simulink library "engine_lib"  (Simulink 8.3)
settings: Solver=ode45  StartTime=0.0  StopTime=10.0  RelTol=1e-3
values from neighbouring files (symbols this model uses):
  engine = class_REVS_engine    [engine_2010_NA.m]    (also in engine_EGRB24_TDS.m)
libraries: general_lib x43, simulink x11, audit_lib x2

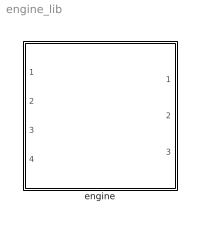
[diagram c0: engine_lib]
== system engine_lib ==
  engine : Subsystem

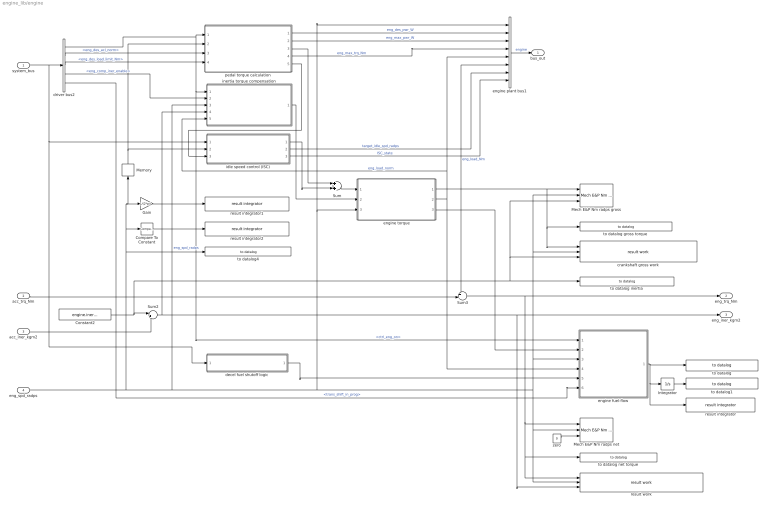
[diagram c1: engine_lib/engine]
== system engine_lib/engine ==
  system_bus : Inport
  acc_trq_Nm : Inport  Port=2
  acc_iner_kgm2 : Inport  Port=3
  eng_spd_radps : Inport  Port=4
  Compare To Constant : simulink/Logic and Bit Operations/Compare To Constant  relop=>  const=0  OutDataTypeStr=boolean  ZeroCross=off
  Constant2 : Constant  Value=engine.inertia_kgm2
  Gain : Gain  Gain=1/(2*pi)
  Integrator : Integrator
  Mech E&P Nm radps gross : audit_lib/Mech E&P Nm radps  base_name=engine.crankshaft_gross  VerboseSignal=REVS.verbose
  Mech E&P Nm radps net : audit_lib/Mech E&P Nm radps  base_name=engine.crankshaft  VerboseSignal=REVS.verbose
  Memory : Memory
  Sum : Sum
  Sum2 : Sum  Inputs=|++
  Sum3 : Sum  Inputs=++|
  crankshaft gross work : general_lib/result work  ResultSignalName=crankshaft_gross_pos_work_kJ
  decel fuel shutoff logic : Subsystem
  driver bus2 : BusSelector  OutputSignals=powertrain.control.ctrl_eng_on,powertrain.trans.ctrl.eng_des_acl_norm,powertrain.trans.ctrl.eng_des_load_limit_Nm,powertrain.trans.ctrl.eng_comp_iner_enable,powertrain.trans.ctrl.core_ctl.trans_shift_in_prog
  engine fuel-flow : Subsystem
  engine plant bus1 : BusCreator  Inputs=8
  engine torque : Subsystem
  idle speed control (ISC) : Subsystem
  inertia torque compensation : Subsystem
  pedal torque calculation : Subsystem
  result integrator : general_lib/result integrator  ResultSignalName=fuel_consumed_g  ResultBaseName=''
  result integrator1 : general_lib/result integrator  ResultSignalName=engine_revolutions  ResultBaseName=''
  result integrator2 : general_lib/result integrator  ResultSignalName=engine_running_time_secs  ResultBaseName=''
  result work : general_lib/result work  ResultSignalName=crankshaft_output_pos_work_kJ
  to datalog : general_lib/to datalog  VarName=engine__fuel_rate_gps  WorkspaceName=datalog__engine__fuel_rate_gps  VerboseLevel=0  VerboseSignal=REVS.verbose
  to datalog gross torque : general_lib/to datalog  VarName=engine__crankshaft_gross_torque_Nm  WorkspaceName=datalog__engine__crankshaft_gross_torque_Nm  VerboseLevel=0  VerboseSignal=REVS.verbose
  to datalog inertia : general_lib/to datalog  VarName=engine__crankshaft_gross_inertia_kgm2  WorkspaceName=datalog__engine__crankshaft_gross_inertia_kgm2  VerboseLevel=0  VerboseSignal=REVS.verbose
  to datalog net torque : general_lib/to datalog  VarName=engine__crankshaft_torque_Nm  WorkspaceName=datalog__engine__crankshaft_torque_Nm  VerboseLevel=0  VerboseSignal=REVS.verbose
  to datalog1 : general_lib/to datalog  VarName=engine__fuel_consumed_g  WorkspaceName=datalog__engine__fuel_consumed_g  VerboseLevel=0  VerboseSignal=REVS.verbose
  to datalog4 : general_lib/to datalog  VarName=engine__crankshaft_speed_radps  WorkspaceName=datalog__engine__crankshaft_speed_radps  VerboseLevel=0  VerboseSignal=REVS.verbose
  zero : Constant  Value=0
  bus_out : Outport
  eng_trq_Nm : Outport  Port=2
  eng_iner_kgm2 : Outport  Port=3
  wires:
  idle speed control (ISC)/2(target_idle_spd_radps) -> engine plant bus1/7  "target_idle_spd_radps"
  decel fuel shutoff logic/1(eng_decel_fuel_cut_disable) -> engine fuel-flow/5(eng_decel_fuel_cut_disable)
  engine torque/3(eng_fuel_trq_Nm) -> engine fuel-flow/2(eng_trq_Nm)
  acc_trq_Nm/1 -> Sum3/2
  pedal torque calculation/2(current_max_pwr_W) -> engine plant bus1/3  "eng_max_pwr_W"
  pedal torque calculation/1(des_pwr_W) -> engine plant bus1/2  "eng_des_pwr_W"
  acc_iner_kgm2/1 -> Sum2/2
  driver bus2/2 -> pedal torque calculation/3(eng_des_acl_norm)  "<eng_des_acl_norm>"
  engine plant bus1/1 -> bus_out/1  "engine"
  pedal torque calculation/3(des_trq_Nm) -> Sum/1
  idle speed control (ISC)/1(trq_out_Nm) -> Sum/2
  Sum/1 -> engine torque/1(eng_slow_trq_Nm)
  system_bus/1 -> decel fuel shutoff logic/1(system_bus), idle speed control (ISC)/1(system_bus), driver bus2/1
  driver bus2/1 -> inertia torque compensation/1(eng_on), engine fuel-flow/1(eng_on), pedal torque calculation/1(eng_on)  "<ctrl_eng_on>"
  Memory/1 -> pedal torque calculation/2(eng_spd_radps), idle speed control (ISC)/2(eng_spd_radps)
  engine torque/2(eng_load_norm) -> engine fuel-flow/4(eng_load_norm), engine plant bus1/5, inertia torque compensation/5(load_norm)  "eng_load_norm"
  Sum2/1 -> result work/3, eng_iner_kgm2/1, inertia torque compensation/4(iner_kgm2)
  driver bus2/4 -> inertia torque compensation/2(comp_iner_enable)  "<eng_comp_iner_enable>"
  driver bus2/3 -> pedal torque calculation/4(eng_des_load_limit_Nm)  "<eng_des_load_limit_Nm>"
  pedal torque calculation/4(current_max_trq_Nm) -> engine plant bus1/4  "eng_max_trq_Nm"
  inertia torque compensation/1(comp_trq_Nm) -> engine torque/2(eng_fast_trq_Nm)
  engine fuel-flow/1(fuel_flow_rate_gps) -> result integrator/1, Integrator/1, to datalog/1
  Integrator/1 -> to datalog1/1
  engine torque/1(eng_load_Nm) -> engine plant bus1/6, Sum3/1, crankshaft gross work/1, to datalog gross torque/1, Mech E&P Nm radps gross/1  "eng_load_Nm"
  Sum3/1 -> result work/1, to datalog net torque/1, Mech E&P Nm radps net/1, eng_trq_Nm/1
  eng_spd_radps/1 -> Memory/1, Gain/1, Compare To Constant/1, to datalog4/1, inertia torque compensation/3(eng_spd_radps), engine plant bus1/1, engine torque/3(eng_spd_radps), engine fuel-flow/3(eng_spd_radps), crankshaft gross work/2, Mech E&P Nm radps gross/2, Mech E&P Nm radps net/2, result work/2  "eng_spd_radps"
  zero/1 -> Mech E&P Nm radps net/3
  Constant2/1 -> to datalog inertia/1, Mech E&P Nm radps gross/3, crankshaft gross work/3, Sum2/1
  driver bus2/5 -> engine fuel-flow/6(shift_in_prog)  "<trans_shift_in_prog>"
  Gain/1 -> result integrator1/1
  Compare To Constant/1 -> result integrator2/1
  pedal torque calculation/5(current_min_trq_Nm) -> idle speed control (ISC)/3(eng_min_trq_Nm)
  idle speed control (ISC)/3(ISC_state) -> engine plant bus1/8  "ISC_state"

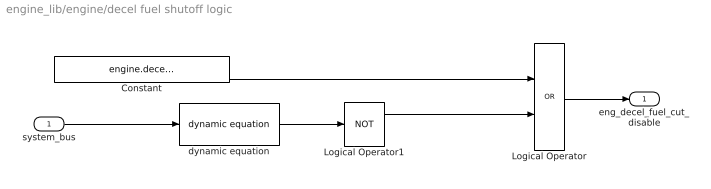
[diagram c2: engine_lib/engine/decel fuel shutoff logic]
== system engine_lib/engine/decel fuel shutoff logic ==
  system_bus : Inport
  Constant : Constant  Value=engine.decel_fuel_shutoff_disabled
  Logical Operator : Logic  Operator=OR  AllPortsSameDT=off  OutDataTypeStr=boolean
  Logical Operator1 : Logic  Operator=NOT  AllPortsSameDT=off  OutDataTypeStr=boolean
  dynamic equation : general_lib/dynamic equation  DynamicExpression=engine.decel_fuel_shutoff_condition  DynamicExpressionEval=1
  eng_decel_fuel_cut_disable : Outport
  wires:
  Logical Operator/1 -> eng_decel_fuel_cut_disable/1
  Constant/1 -> Logical Operator/1
  system_bus/1 -> dynamic equation/1
  dynamic equation/1 -> Logical Operator1/1
  Logical Operator1/1 -> Logical Operator/2

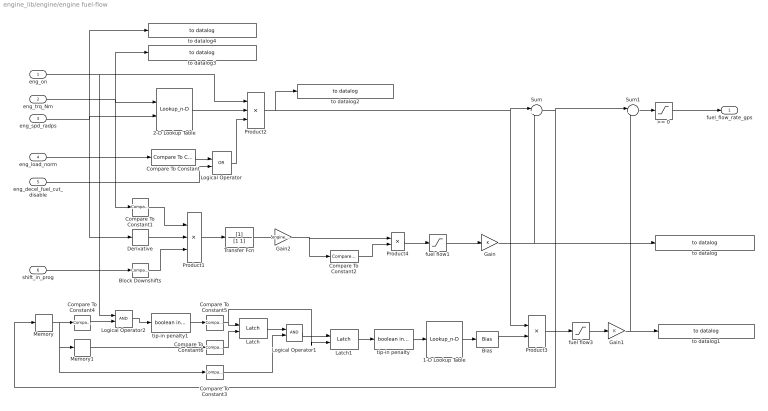
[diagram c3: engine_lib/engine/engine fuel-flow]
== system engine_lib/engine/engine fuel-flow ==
  eng_on : Inport
  eng_trq_Nm : Inport  Port=2
  eng_spd_radps : Inport  Port=3
  eng_load_norm : Inport  Port=4
  eng_decel_fuel_cut_disable : Inport  Port=5
  shift_in_prog : Inport  Port=6
  1-D Lookup Table : Lookup_n-D  NumberOfTableDimensions=1  BreakpointsForDimension1=engine.refuel_profile_time_secs  IndexSearchMethod=Linear search  BeginIndexSearchUsingPreviousIndexResult=on  Table=engine.refuel_profile_mult  ExtrapMethod=Clip  RndMeth=Simplest
  2-D Lookup Table : Lookup_n-D  BreakpointsForDimension1=engine.fuel_map_torque_Nm  BreakpointsForDimension2=engine.fuel_map_speed_radps  IndexSearchMethod=Linear search  BeginIndexSearchUsingPreviousIndexResult=on  Table=engine.fuel_map_gps  ExtrapMethod=Clip  UseLastTableValue=on  RndMeth=Simplest
  >= 0 : Saturate  UpperLimit=Inf  LowerLimit=0  ZeroCross=off
  Bias : Bias  Bias=-1
  Block Downshifts : simulink/Logic and Bit Operations/Compare To Constant  relop=>=  const=0  OutDataTypeStr=boolean  ZeroCross=off
  Compare To Constant : simulink/Logic and Bit Operations/Compare To Constant  relop=>=  const=eps  OutDataTypeStr=boolean  ZeroCross=off
  Compare To Constant1 : simulink/Logic and Bit Operations/Compare To Constant  relop=>  const=0  OutDataTypeStr=boolean  ZeroCross=off
  Compare To Constant2 : simulink/Logic and Bit Operations/Compare To Constant  relop=>=  const=engine.acceleration_penalty_squelch_gps  OutDataTypeStr=boolean  ZeroCross=off
  Compare To Constant3 : simulink/Logic and Bit Operations/Compare To Constant  relop=~=  const=0  OutDataTypeStr=boolean  ZeroCross=off
  Compare To Constant4 : simulink/Logic and Bit Operations/Compare To Constant  relop=<=  const=0  OutDataTypeStr=boolean  ZeroCross=off
  Compare To Constant5 : simulink/Logic and Bit Operations/Compare To Constant  relop=>=  const=engine.refuel_min_defuel_duration_secs  OutDataTypeStr=boolean  ZeroCross=off
  Compare To Constant6 : simulink/Logic and Bit Operations/Compare To Constant  relop=~=  const=0  OutDataTypeStr=boolean  ZeroCross=off
  Derivative : Derivative
  Gain : Gain
  Gain1 : Gain
  Gain2 : Gain  Gain=engine.acceleration_penalty_gpradps2
  Latch : general_lib/Latch  tb=Off  InitialCondition=0
  Latch1 : general_lib/Latch  tb=Off  InitialCondition=0
  Logical Operator : Logic  Operator=OR  AllPortsSameDT=off  OutDataTypeStr=boolean
  Logical Operator1 : Logic  AllPortsSameDT=off  OutDataTypeStr=boolean
  Logical Operator2 : Logic  AllPortsSameDT=off  OutDataTypeStr=boolean
  Memory : Memory
  Memory1 : Memory
  Product1 : Product  Inputs=3
  Product2 : Product  Inputs=3
  Product3 : Product
  Product4 : Product
  Sum : Sum  Inputs=|++
  Sum1 : Sum  Inputs=|++
  Transfer Fcn : TransferFcn  Denominator=[1 1]
  fuel flow1 : Saturate  UpperLimit=inf  LowerLimit=0  ZeroCross=off
  fuel flow3 : Saturate  UpperLimit=engine.refuel_limit_gps  LowerLimit=0  ZeroCross=off
  tip-in penalty : general_lib/boolean integrator  UpperSaturationLimit=Inf  Normalize=off
  tip-in penalty1 : general_lib/boolean integrator  UpperSaturationLimit=Inf  Normalize=off
  to datalog : general_lib/to datalog  VarName=engine__accel_penalty_gps  WorkspaceName=datalog__engine__accel_penalty_gps  VerboseLevel=1  VerboseSignal=REVS.verbose
  to datalog1 : general_lib/to datalog  VarName=engine__tipin_penalty_gps  WorkspaceName=datalog__engine__tipin_penalty_gps  VerboseLevel=1  VerboseSignal=REVS.verbose
  to datalog2 : general_lib/to datalog  VarName=engine__base_fuel_rate_gps  WorkspaceName=datalog__engine__base_fuel_rate_gps  VerboseLevel=1  VerboseSignal=REVS.verbose
  to datalog3 : general_lib/to datalog  VarName=engine__twoD_eng_trq_Nm  WorkspaceName=datalog__engine__twoD_eng_trq_Nm  VerboseLevel=1  VerboseSignal=REVS.verbose
  to datalog4 : general_lib/to datalog  VarName=engine__twoD_eng_spd_radps  WorkspaceName=datalog__engine__twoD_eng_spd_radps  VerboseLevel=1  VerboseSignal=REVS.verbose
  fuel_flow_rate_gps : Outport
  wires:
  eng_decel_fuel_cut_disable/1 -> Logical Operator/2
  eng_load_norm/1 -> Compare To Constant/1
  eng_on/1 -> Logical Operator2/1, Product2/1
  2-D Lookup Table/1 -> Product2/2
  Compare To Constant/1 -> Logical Operator/1
  Logical Operator/1 -> Product2/3
  >= 0/1 -> fuel_flow_rate_gps/1
  eng_spd_radps/1 -> to datalog4/1, Derivative/1, 2-D Lookup Table/2
  eng_trq_Nm/1 -> 2-D Lookup Table/1, to datalog3/1, Compare To Constant1/1
  Product2/1 -> Sum/1, Product3/1, to datalog2/1
  Compare To Constant1/1 -> Product1/1
  tip-in penalty/1 -> 1-D Lookup Table/1
  1-D Lookup Table/1 -> Bias/1
  Memory/1 -> Compare To Constant4/1, Memory1/1, Compare To Constant3/1
  Compare To Constant4/1 -> Logical Operator2/2
  tip-in penalty1/1 -> Compare To Constant5/1
  Compare To Constant5/1 -> Latch1/2, Latch/1
  Compare To Constant6/1 -> Latch/2
  Memory1/1 -> Compare To Constant6/1
  Latch/1 -> Logical Operator1/1
  Compare To Constant3/1 -> Logical Operator1/2
  Logical Operator1/1 -> Latch1/1
  Latch1/1 -> tip-in penalty/1
  Sum1/1 -> >= 0/1
  Product3/1 -> fuel flow3/1
  fuel flow3/1 -> Gain1/1
  Gain/1 -> to datalog/1, Sum/2
  Gain1/1 -> to datalog1/1, Sum1/2
  fuel flow1/1 -> Gain/1
  Bias/1 -> Product3/2
  Sum/1 -> Sum1/1, Memory/1
  shift_in_prog/1 -> Block Downshifts/1
  Block Downshifts/1 -> Product1/3
  Product4/1 -> fuel flow1/1
  Derivative/1 -> Product1/2
  Product1/1 -> Transfer Fcn/1
  Transfer Fcn/1 -> Gain2/1
  Gain2/1 -> Product4/1, Compare To Constant2/1
  Compare To Constant2/1 -> Product4/2
  Logical Operator2/1 -> tip-in penalty1/1

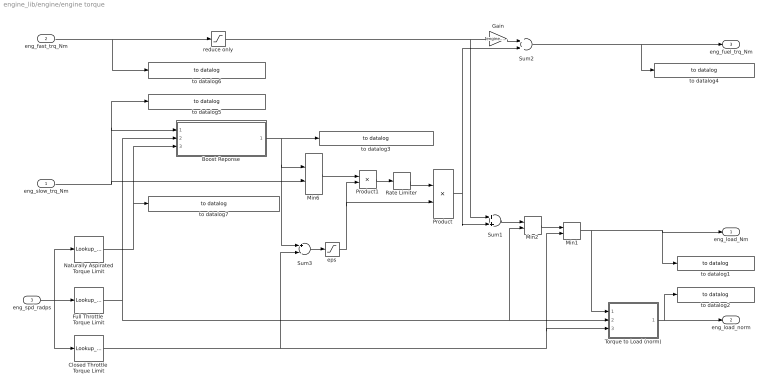
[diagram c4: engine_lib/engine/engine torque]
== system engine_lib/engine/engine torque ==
  eng_slow_trq_Nm : Inport
  eng_fast_trq_Nm : Inport  Port=2
  eng_spd_radps : Inport  Port=3
  Boost Reponse : Subsystem
  Closed Throttle  Torque Limit : Lookup_n-D  NumberOfTableDimensions=1  BreakpointsForDimension1=engine.closed_throttle_speed_radps  BeginIndexSearchUsingPreviousIndexResult=on  Table=engine.closed_throttle_torque_Nm  ExtrapMethod=Clip  UseLastTableValue=on  RndMeth=Simplest
  Full Throttle  Torque Limit : Lookup_n-D  NumberOfTableDimensions=1  BreakpointsForDimension1=engine.full_throttle_speed_radps  BeginIndexSearchUsingPreviousIndexResult=on  Table=engine.full_throttle_torque_Nm  ExtrapMethod=Clip  UseLastTableValue=on  RndMeth=Simplest
  Gain : Gain  Gain=engine.fast_torque_fuel_adjust_norm
  Min1 : MinMax  Function=max  Inputs=2  ZeroCross=off
  Min2 : MinMax  Inputs=2  ZeroCross=off
  Min6 : MinMax  Inputs=2  ZeroCross=off
  Naturally Aspirated Torque Limit : Lookup_n-D  NumberOfTableDimensions=1  BreakpointsForDimension1=engine.naturally_aspirated_speed_radps  IndexSearchMethod=Linear search  BeginIndexSearchUsingPreviousIndexResult=on  Table=engine.naturally_aspirated_torque_Nm  ExtrapMethod=Clip  UseLastTableValue=on  RndMeth=Simplest
  Product : Product
  Product1 : Product  Inputs=*/
  Rate Limiter : RateLimiter  RisingSlewLimit=1/engine.throttle_duration_sec  FallingSlewLimit=-1/engine.throttle_duration_sec  SampleTimeMode=inherited
  Sum1 : Sum
  Sum2 : Sum
  Sum3 : Sum  Inputs=+-
  Torque to Load (norm) : Subsystem
  eps : Saturate  UpperLimit=inf  LowerLimit=eps  ZeroCross=off
  reduce only : Saturate  UpperLimit=0  LowerLimit=-inf  ZeroCross=off
  to datalog1 : general_lib/to datalog  VarName=engine__load_Nm  WorkspaceName=datalog__engine__load_Nm  VerboseLevel=1  VerboseSignal=REVS.verbose
  to datalog2 : general_lib/to datalog  VarName=engine__load_norm  WorkspaceName=datalog__engine__load_norm  VerboseLevel=1  VerboseSignal=REVS.verbose
  to datalog3 : general_lib/to datalog  VarName=engine__available_torque_Nm  WorkspaceName=datalog__engine__available_torque_Nm  VerboseLevel=2  VerboseSignal=REVS.verbose
  to datalog4 : general_lib/to datalog  VarName=engine__fueling_torque_Nm  WorkspaceName=datalog__engine__fueling_torque_Nm  VerboseLevel=1  VerboseSignal=REVS.verbose
  to datalog5 : general_lib/to datalog  VarName=engine.slow_target_torque_Nm  WorkspaceName=datalog__engine__slow_target_torque_Nm  VerboseLevel=1  VerboseSignal=REVS.verbose
  to datalog6 : general_lib/to datalog  VarName=engine.fast_target_torque_Nm  WorkspaceName=datalog__engine__fast_target_torque_Nm  VerboseLevel=1  VerboseSignal=REVS.verbose
  to datalog7 : general_lib/to datalog  VarName=engine.naturally_aspirated_torque_Nm  WorkspaceName=datalog__engine__naturally_aspirated_torque_Nm  VerboseLevel=1  VerboseSignal=REVS.verbose
  eng_load_Nm : Outport
  eng_load_norm : Outport  Port=2
  eng_fuel_trq_Nm : Outport  Port=3
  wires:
  Torque to Load (norm)/1(load_norm) -> eng_load_norm/1, to datalog2/1
  Closed Throttle  Torque Limit/1 -> Torque to Load (norm)/3(min), Min1/2, Sum3/2
  Full Throttle  Torque Limit/1 -> Torque to Load (norm)/2(max), Min2/2, Boost Reponse/2(max_trq_Nm)
  Naturally Aspirated Torque Limit/1 -> Boost Reponse/3(nat_asp_trq_Nm), to datalog7/1
  eng_slow_trq_Nm/1 -> Min6/2, to datalog5/1, Boost Reponse/1(target_trq_Nm)
  Product/1 -> Sum1/2, Sum2/2
  Gain/1 -> Sum2/1
  Sum2/1 -> eng_fuel_trq_Nm/1, to datalog4/1
  Sum1/1 -> Min2/1
  reduce only/1 -> Gain/1, Sum1/1
  eng_fast_trq_Nm/1 -> reduce only/1, to datalog6/1
  eng_spd_radps/1 -> Closed Throttle  Torque Limit/1, Naturally Aspirated Torque Limit/1, Full Throttle  Torque Limit/1
  Min1/1 -> eng_load_Nm/1, to datalog1/1, Torque to Load (norm)/1(torque)
  Min2/1 -> Min1/1
  Min6/1 -> Product1/1
  Product1/1 -> Rate Limiter/1
  Rate Limiter/1 -> Product/1
  Boost Reponse/1(trq_limit_Nm) -> Sum3/1, Min6/1, to datalog3/1
  Sum3/1 -> eps/1
  eps/1 -> Product/2, Product1/2

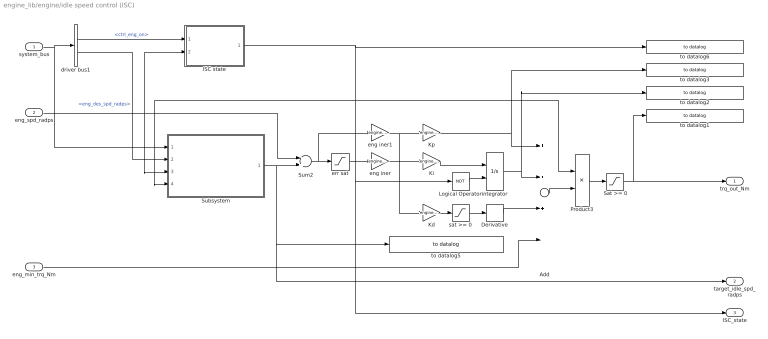
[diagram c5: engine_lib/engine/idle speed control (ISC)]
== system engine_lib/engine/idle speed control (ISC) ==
  system_bus : Inport
  eng_spd_radps : Inport  Port=2
  eng_min_trq_Nm : Inport  Port=3
  " Sat >= 0" : Saturate  UpperLimit=inf  LowerLimit=0  ZeroCross=off
  Add : Sum  Inputs=+++-
  Derivative : Derivative
  ISC state : Subsystem
  Integrator : Integrator  ExternalReset=level  LimitOutput=on  UpperSaturationLimit=Inf  LowerSaturationLimit=0
  Kd : Gain  Gain=engine.idle_control_Kd
  Ki : Gain  Gain=engine.idle_control_Ki
  Kp : Gain  Gain=engine.idle_control_Kp
  Logical Operator : Logic  Operator=NOT  AllPortsSameDT=off  OutDataTypeStr=boolean
  Product3 : Product
  Subsystem : Subsystem
  Sum2 : Sum  Inputs=-+
  driver bus1 : BusSelector  OutputSignals=powertrain.control.ctrl_eng_on,powertrain.trans.ctrl.eng_des_spd_radps
  eng iner : Gain  Gain=engine.inertia_kgm2
  eng iner1 : Gain  Gain=engine.inertia_kgm2
  err sat : Saturate  UpperLimit=2.5  LowerLimit=-Inf  ZeroCross=off
  sat >= 0 : Saturate  UpperLimit=Inf  LowerLimit=0  ZeroCross=off
  to datalog1 : general_lib/to datalog  VarName=engine__ISC_torque_Nm  WorkspaceName=datalog__engine__ISC_torque_Nm  VerboseLevel=1  VerboseSignal=REVS.verbose
  to datalog2 : general_lib/to datalog  VarName=engine__ISC_Ki_torque_Nm  WorkspaceName=datalog__engine__ISC_Ki_torque_Nm  VerboseLevel=3  VerboseSignal=REVS.verbose
  to datalog3 : general_lib/to datalog  VarName=engine__ISC_Kp_torque_Nm  WorkspaceName=datalog__engine__ISC_Kp_torque_Nm  VerboseLevel=3  VerboseSignal=REVS.verbose
  to datalog5 : general_lib/to datalog  VarName=engine__ISC_target_speed_radps  WorkspaceName=datalog__engine__ISC_target_speed_radps  VerboseLevel=1  VerboseSignal=REVS.verbose
  to datalog6 : general_lib/to datalog  VarName=engine__ISC_state  WorkspaceName=datalog__engine__ISC_state  VerboseLevel=3  VerboseSignal=REVS.verbose
  trq_out_Nm : Outport
  target_idle_spd_radps : Outport  Port=2
  ISC_state : Outport  Port=3
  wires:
  driver bus1/1 -> ISC state/1(eng_on)  "<ctrl_eng_on>"
  system_bus/1 -> Subsystem/1(system_bus), driver bus1/1
  Logical Operator/1 -> Integrator/2
  Product3/1 -> " Sat >= 0"/1
  Kd/1 -> sat >= 0/1
  Add/1 -> Product3/2
  Ki/1 -> Integrator/1
  Derivative/1 -> Add/3
  eng_spd_radps/1 -> Subsystem/3(eng_spd_radps), Sum2/1, ISC state/2(eng_spd_radps)
  " Sat >= 0"/1 -> to datalog1/1, trq_out_Nm/1
  Kp/1 -> to datalog3/1, Add/1
  Integrator/1 -> to datalog2/1, Add/2
  Sum2/1 -> eng iner1/1, err sat/1
  eng iner/1 -> Ki/1
  Subsystem/1(target_idle_spd_radps) -> Sum2/2, to datalog5/1, target_idle_spd_radps/1
  driver bus1/2 -> Subsystem/2(eng_des_spd_radps)  "<eng_des_spd_radps>"
  eng_min_trq_Nm/1 -> Add/4
  ISC state/1(state) -> to datalog6/1, Subsystem/4(ISC_state), Product3/1, ISC_state/1, Logical Operator/1
  sat >= 0/1 -> Derivative/1
  err sat/1 -> eng iner/1
  eng iner1/1 -> Kd/1, Kp/1

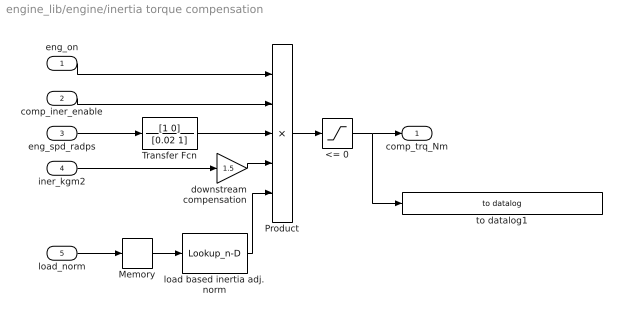
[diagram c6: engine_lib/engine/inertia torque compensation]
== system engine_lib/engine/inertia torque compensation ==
  eng_on : Inport
  comp_iner_enable : Inport  Port=2
  eng_spd_radps : Inport  Port=3
  iner_kgm2 : Inport  Port=4
  load_norm : Inport  Port=5
  <= 0 : Saturate  UpperLimit=0  LowerLimit=-Inf  ZeroCross=off
  Memory : Memory
  Product : Product  Inputs=5
  Transfer Fcn : TransferFcn  Numerator=[1 0]  Denominator=[0.02 1]
  downstream compensation : Gain  Gain=1.5
  load based inertia adj. norm : Lookup_n-D  NumberOfTableDimensions=1  BreakpointsForDimension1=[0, 0.65, 0.90, 1.0]  Table=[1.0, 1.0, 0.0, 0.0]  InternalRulePriority=Speed  RndMeth=Simplest
  to datalog1 : general_lib/to datalog  VarName=engine.inertia_comp_torque_Nm  WorkspaceName=datalog__engine__inertia_comp_torque_Nm  VerboseLevel=1  VerboseSignal=REVS.verbose
  comp_trq_Nm : Outport
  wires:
  comp_iner_enable/1 -> Product/2
  downstream compensation/1 -> Product/4
  Transfer Fcn/1 -> Product/3
  eng_spd_radps/1 -> Transfer Fcn/1
  iner_kgm2/1 -> downstream compensation/1
  <= 0/1 -> to datalog1/1, comp_trq_Nm/1
  eng_on/1 -> Product/1
  load_norm/1 -> Memory/1
  Memory/1 -> load based inertia adj. norm/1
  load based inertia adj. norm/1 -> Product/5
  Product/1 -> <= 0/1

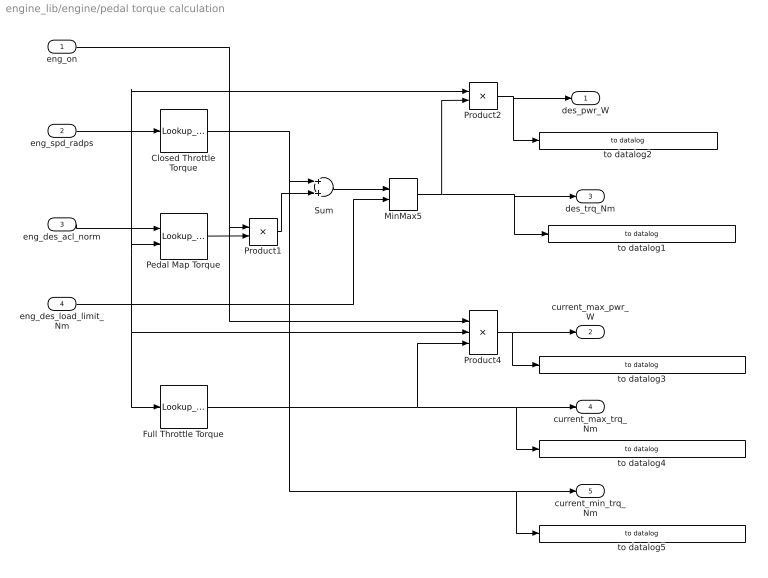
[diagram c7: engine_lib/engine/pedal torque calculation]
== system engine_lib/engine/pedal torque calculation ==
  eng_on : Inport
  eng_spd_radps : Inport  Port=2
  eng_des_acl_norm : Inport  Port=3
  eng_des_load_limit_Nm : Inport  Port=4
  Closed Throttle Torque : Lookup_n-D  NumberOfTableDimensions=1  BreakpointsForDimension1=engine.closed_throttle_speed_radps  BeginIndexSearchUsingPreviousIndexResult=on  Table=engine.closed_throttle_torque_Nm  ExtrapMethod=Clip  UseLastTableValue=on  RndMeth=Simplest
  Full Throttle Torque : Lookup_n-D  NumberOfTableDimensions=1  BreakpointsForDimension1=engine.full_throttle_speed_radps  BeginIndexSearchUsingPreviousIndexResult=on  Table=engine.full_throttle_torque_Nm  ExtrapMethod=Clip  UseLastTableValue=on  RndMeth=Simplest
  MinMax5 : MinMax  Inputs=2  ZeroCross=off
  Pedal Map Torque : Lookup_n-D  BreakpointsForDimension1=engine.pedal_map_pedal_norm  BreakpointsForDimension2=engine.pedal_map_speed_radps  BeginIndexSearchUsingPreviousIndexResult=on  Table=engine.pedal_map_Nm  RndMeth=Simplest
  Product1 : Product
  Product2 : Product
  Product4 : Product  Inputs=3
  Sum : Sum
  to datalog1 : general_lib/to datalog  VarName=engine__accel_pedal_torque_Nm  WorkspaceName=datalog__engine__accel_pedal_torque_Nm  VerboseLevel=1  VerboseSignal=REVS.verbose
  to datalog2 : general_lib/to datalog  VarName=engine__accel_pedal_power_W  WorkspaceName=datalog__engine__accel_pedal_power_W  VerboseLevel=1  VerboseSignal=REVS.verbose
  to datalog3 : general_lib/to datalog  VarName=engine__current_available_power_W  WorkspaceName=datalog__engine__current_available_power_W  VerboseLevel=1  VerboseSignal=REVS.verbose
  to datalog4 : general_lib/to datalog  VarName=engine__current_available_torque_Nm  WorkspaceName=datalog__engine__current_available_torque_Nm  VerboseLevel=1  VerboseSignal=REVS.verbose
  to datalog5 : general_lib/to datalog  VarName=engine__current_min_torque_Nm  WorkspaceName=datalog__engine__current_min_torque_Nm  VerboseLevel=1  VerboseSignal=REVS.verbose
  des_pwr_W : Outport
  current_max_pwr_W : Outport  Port=2
  des_trq_Nm : Outport  Port=3
  current_max_trq_Nm : Outport  Port=4
  current_min_trq_Nm : Outport  Port=5
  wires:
  eng_des_acl_norm/1 -> Pedal Map Torque/1
  Sum/1 -> MinMax5/1
  Product1/1 -> Sum/2
  Closed Throttle Torque/1 -> to datalog5/1, current_min_trq_Nm/1, Sum/1
  eng_on/1 -> Product1/1, Product4/1
  MinMax5/1 -> Product2/2, des_trq_Nm/1, to datalog1/1
  Product2/1 -> des_pwr_W/1, to datalog2/1
  eng_spd_radps/1 -> Pedal Map Torque/2, Product4/2, Full Throttle Torque/1, Closed Throttle Torque/1, Product2/1
  Product4/1 -> to datalog3/1, current_max_pwr_W/1
  Full Throttle Torque/1 -> Product4/3, to datalog4/1, current_max_trq_Nm/1
  eng_des_load_limit_Nm/1 -> MinMax5/2
  Pedal Map Torque/1 -> Product1/2

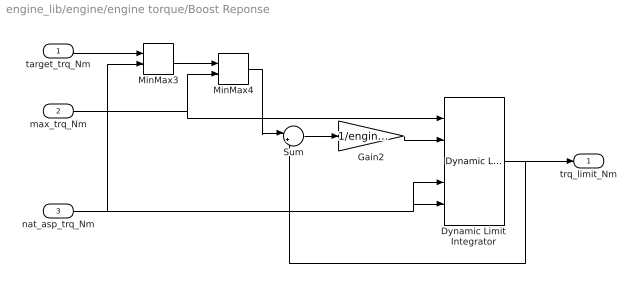
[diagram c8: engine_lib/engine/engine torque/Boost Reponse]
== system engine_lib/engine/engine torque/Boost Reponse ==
  target_trq_Nm : Inport
  max_trq_Nm : Inport  Port=2
  nat_asp_trq_Nm : Inport  Port=3
  Dynamic Limit Integrator : general_lib/Dynamic Limit Integrator
  Gain2 : Gain  Gain=1/engine.boost_time_constant_sec
  MinMax3 : MinMax  Function=max  Inputs=2  ZeroCross=off
  MinMax4 : MinMax  Inputs=2  ZeroCross=off
  Sum : Sum  Inputs=|+-
  trq_limit_Nm : Outport
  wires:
  target_trq_Nm/1 -> MinMax3/1
  max_trq_Nm/1 -> MinMax4/2, Dynamic Limit Integrator/1
  nat_asp_trq_Nm/1 -> MinMax3/2, Dynamic Limit Integrator/4, Dynamic Limit Integrator/5
  Gain2/1 -> Dynamic Limit Integrator/2
  MinMax4/1 -> Sum/1
  Sum/1 -> Gain2/1
  MinMax3/1 -> MinMax4/1
  Dynamic Limit Integrator/1 -> trq_limit_Nm/1, Sum/2

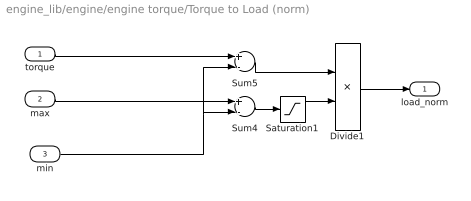
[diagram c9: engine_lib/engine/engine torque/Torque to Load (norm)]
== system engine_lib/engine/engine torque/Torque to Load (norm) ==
  torque : Inport
  max : Inport  Port=2
  min : Inport  Port=3
  Divide1 : Product  Inputs=*/
  Saturation1 : Saturate  UpperLimit=Inf  LowerLimit=1  ZeroCross=off
  Sum4 : Sum  Inputs=+-
  Sum5 : Sum  Inputs=+-
  load_norm : Outport
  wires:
  Saturation1/1 -> Divide1/2
  Sum4/1 -> Saturation1/1
  torque/1 -> Sum5/1
  Sum5/1 -> Divide1/1
  Divide1/1 -> load_norm/1
  min/1 -> Sum4/2, Sum5/2
  max/1 -> Sum4/1

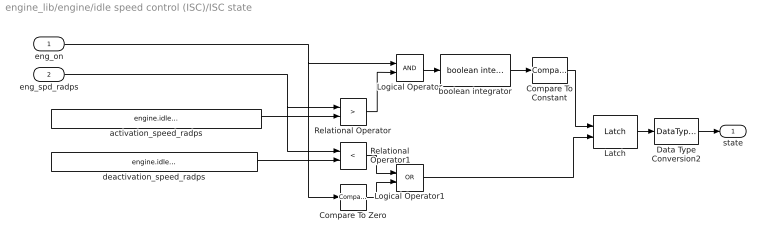
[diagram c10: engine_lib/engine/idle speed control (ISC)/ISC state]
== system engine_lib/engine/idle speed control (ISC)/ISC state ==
  eng_on : Inport
  eng_spd_radps : Inport  Port=2
  Compare To Constant : simulink/Logic and Bit Operations/Compare To Constant  relop=>  const=0.5  OutDataTypeStr=boolean
  Compare To Zero : simulink/Logic and Bit Operations/Compare To Zero  relop===  OutDataTypeStr=boolean
  Data Type Conversion2 : DataTypeConversion
  Latch : general_lib/Latch  tb=Off  InitialCondition=0
  Logical Operator : Logic  AllPortsSameDT=off  OutDataTypeStr=boolean
  Logical Operator1 : Logic  Operator=OR  AllPortsSameDT=off  OutDataTypeStr=boolean
  Relational Operator : RelationalOperator  Operator=>  OutDataTypeStr=boolean
  Relational Operator1 : RelationalOperator  Operator=<  OutDataTypeStr=boolean
  activation_speed_radps : Constant  Value=engine.idle_control_activation_speed_radps
  boolean integrator : general_lib/boolean integrator  UpperSaturationLimit=1  Normalize=off
  deactivation_speed_radps : Constant  Value=engine.idle_control_deactivation_speed_radps
  state : Outport
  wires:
  Relational Operator/1 -> Logical Operator/2
  boolean integrator/1 -> Compare To Constant/1
  eng_spd_radps/1 -> Relational Operator1/1, Relational Operator/1
  activation_speed_radps/1 -> Relational Operator/2
  Logical Operator1/1 -> Latch/2
  Compare To Constant/1 -> Latch/1
  deactivation_speed_radps/1 -> Relational Operator1/2
  Latch/1 -> Data Type Conversion2/1
  Data Type Conversion2/1 -> state/1
  Logical Operator/1 -> boolean integrator/1
  eng_on/1 -> Compare To Zero/1, Logical Operator/1
  Relational Operator1/1 -> Logical Operator1/1
  Compare To Zero/1 -> Logical Operator1/2

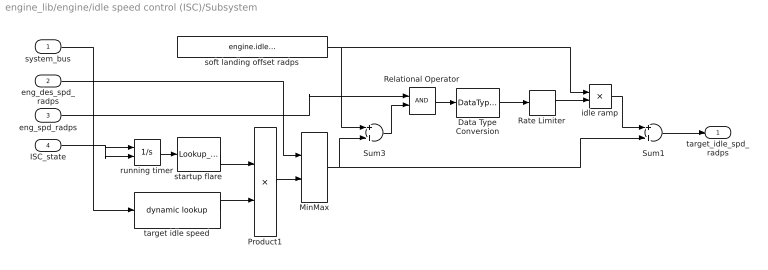
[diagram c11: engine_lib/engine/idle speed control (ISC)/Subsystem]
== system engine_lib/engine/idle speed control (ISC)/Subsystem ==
  system_bus : Inport
  eng_des_spd_radps : Inport  Port=2
  eng_spd_radps : Inport  Port=3
  ISC_state : Inport  Port=4
  Data Type Conversion : DataTypeConversion
  MinMax : MinMax  Function=max  Inputs=2
  Product1 : Product
  Rate Limiter : RateLimiter  RisingSlewLimit=1/engine.idle_control_ramp_time_secs  FallingSlewLimit=-1/engine.idle_control_ramp_time_secs  SampleTimeMode=inherited
  Relational Operator : RelationalOperator  OutDataTypeStr=boolean
  Sum1 : Sum
  Sum3 : Sum
  idle ramp : Product
  running timer : Integrator  ExternalReset=falling
  soft landing offset radps : Constant  Value=engine.idle_control_ramp_radps
  startup flare : Lookup_n-D  NumberOfTableDimensions=1  BreakpointsForDimension1=[0 0.5 1.25 2.25 3.0 3.5]  IndexSearchMethod=Linear search  Table="[0.5 1.1 1.2 1.2  1.1 1.0]"  InterpMethod=Cubic spline  ExtrapMethod=Clip  RndMeth=Simplest
  target idle speed : general_lib/dynamic lookup  LookupStructure=engine.idle_speed_radps  InterpMethod=Linear  ExtrapMethod=Linear  DiagnosticForOutOfRangeInput=None  IndexSearchMethod=Linear search  BeginIndexSearchUsingPreviousIndexResult=on  SupportTunableTableSize=off  LookupStructureEval=|
      | LookupStructure =
      | 
      |      []
  target_idle_spd_radps : Outport
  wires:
  system_bus/1 -> target idle speed/1
  eng_spd_radps/1 -> Relational Operator/1
  ISC_state/1 -> running timer/2, running timer/1
  startup flare/1 -> Product1/1
  eng_des_spd_radps/1 -> MinMax/1
  target idle speed/1 -> Product1/2
  MinMax/1 -> Sum1/2, Sum3/2
  Product1/1 -> MinMax/2
  running timer/1 -> startup flare/1
  Relational Operator/1 -> Data Type Conversion/1
  soft landing offset radps/1 -> idle ramp/1, Sum3/1
  Rate Limiter/1 -> idle ramp/2
  Sum3/1 -> Relational Operator/2
  idle ramp/1 -> Sum1/1
  Data Type Conversion/1 -> Rate Limiter/1
  Sum1/1 -> target_idle_spd_radps/1
